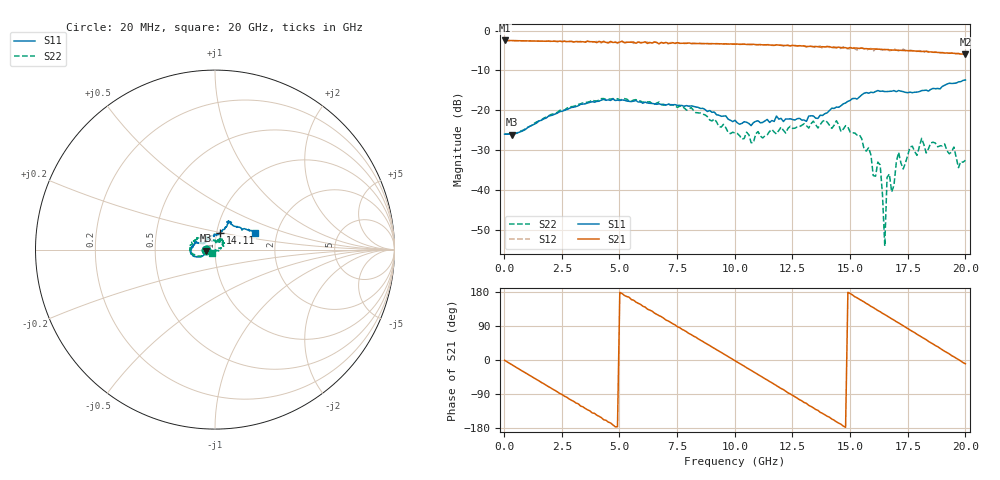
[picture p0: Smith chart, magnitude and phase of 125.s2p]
!Agilent Technologies,N5230A,US43500223,A.07.50.48
!Agilent N5230A: A.07.50.48
!Date: Thursday, September 17, 2015 19:51:00
!Correction: S11(Full 2 Port(1,2))
!S21(Full 2 Port(1,2))
!S12(Full 2 Port(1,2))
!S22(Full 2 Port(1,2))
!S2P File: Measurements: S11, S21, S12, S22:
# Hz S  dB  R 50
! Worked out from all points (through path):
!   201 points, 20 MHz to 20 GHz, reference 50 ohm
!   highest |S21| = -2.47 dB at 20 MHz (marker M1); lowest = -6.0 dB at 20 GHz (marker M2)
!   group delay of S21, straight-line fit = 101 ps
!   lowest |S11| = -26.1 dB at 319.7 MHz (marker M3), VSWR 1.10, Z = 45.3 - j0.498 ohm
!   |S11| at or under -10 dB: start of sweep to end of sweep
!   |S22| runs from -54.1 to -17.0 dB; largest |S21 - S12| = 0.057
!   S11 on the Smith chart (normalised r, x): 20 MHz: 0.90, +0.00; 14.11 GHz: 1.04, +0.20; 20 GHz: 1.54, +0.30
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2e7  -25.96 179.5  -2.47 -0.8  -2.47 -0.9  -25.95 179.4
3.197e8  -26.05 -173.7  -2.51 -12.0  -2.52 -11.9  -25.84 -173.1
1.9181e9  -21.48 -152.8  -2.61 -70.2  -2.62 -70.3  -21.40 -154.2
3.4166e9  -18.43 -161.8  -2.78 -123.6  -2.98 -123.6  -18.12 -166.5
5.1149e9  -17.39 -178.5  -2.65 175.3  -2.73 175.8  -17.26 171.2
6.7133e9  -18.34 166.7  -3.33 117.2  -3.24 117.1  -17.91 151.7
8.012e9  -18.96 158.9  -3.10 70.0  -3.09 70.8  -19.65 139.6
1.001e10  -22.49 150.0  -3.38 -1.9  -3.33 -1.3  -25.68 98.7
1.19081e10  -22.18 121.0  -3.65 -71.4  -3.62 -71.6  -25.08 65.5
1.34066e10  -21.41 86.1  -4.02 -126.2  -4.06 -127.0  -22.71 54.9
1.41059e10  -20.04 72.1  -4.02 -151.0  -4.22 -152.9  -23.73 50.4
1.54046e10  -16.64 63.1  -4.47 160.1  -4.31 164.4  -26.11 35.2
1.6004e10  -15.55 66.8  -4.60 138.4  -5.19 138.6  -36.34 25.4
1.63037e10  -15.22 63.8  -4.68 127.4  -4.72 126.3  -33.66 -21.2
1.65035e10  -15.29 62.7  -4.77 120.0  -4.72 122.2  -54.05 -65.4
1.66034e10  -15.28 61.6  -4.76 116.2  -4.43 116.6  -36.79 -85.5
1.67033e10  -15.23 64.1  -4.85 112.1  -5.05 113.1  -35.96 -84.7
1.68032e10  -15.19 61.6  -4.86 108.7  -4.91 110.9  -40.44 -68.8
1.71029e10  -15.02 58.9  -4.92 97.9  -5.08 99.8  -30.51 -126.2
1.73027e10  -15.30 59.5  -4.97 90.4  -4.63 92.0  -34.69 -114.9
1.81019e10  -15.04 46.5  -5.23 60.9  -5.14 61.4  -27.01 -130.7
2e10  -12.38 22.2  -5.98 -9.9  -5.91 -8.0  -32.50 -132.7
